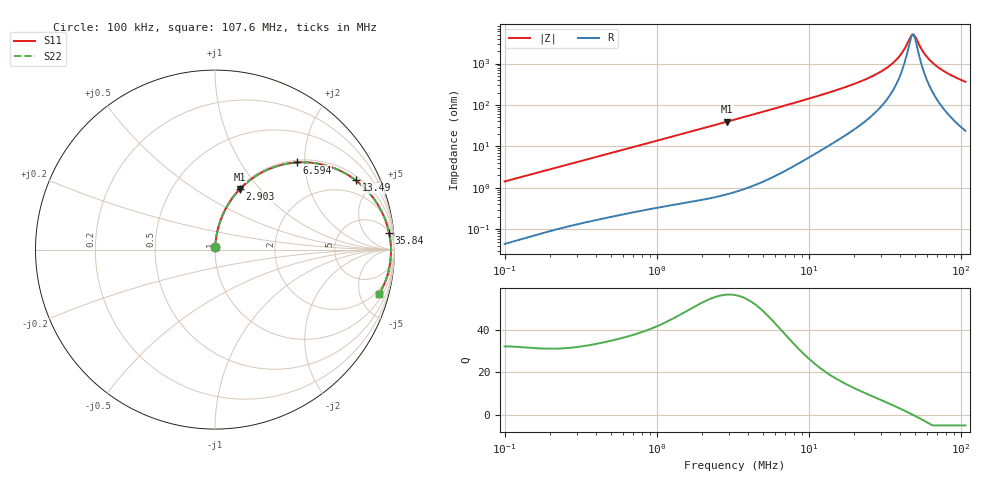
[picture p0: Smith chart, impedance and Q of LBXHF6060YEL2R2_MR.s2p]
! LBXHF6060YEL2R2_MR  S-PARAMETER MODEL  ( General Type )
! Model Generated by TAIYO YUDEN Corporation (http://www.ty-top.com)
! Version 1.0
! TAIYO YUDEN Control No. 200120NI43SB-FBB
! Copyright(c) 2020 TAIYO YUDEN CO.,LTD. All Rights Reserved.
! Product Description (link to TY-COMPAS)
! https://ds.yuden.co.jp/TYCOMPAS/or/detail?pn=LBXHF6060YEL2R2NMR&u=M
! Products Name : Inductors
! Characteristics :
!  Inductance : 2.2 uH , SRF(min) : 36 MHz , DC Resistance(max) : 0.023 Ohm
!  Rated Current : Saturation :8500 mA , Temp Rise : 3000 mA
!  Case Size : 6.0 x 6.0 / 0.236 x 0.236 [mm/inch] , Thickness : 4.5 / 0.177 [mm/inch]
!  (Conditions: Temperature = 25 degC , DC Bias Current/Voltage = 0A / 0V)
! External Node Assignments :
!  1  o---GGG---o  2
! GND o---------o GND
! Frequency Range : 0.1MHz  -  107.617193MHz  [ 402 STEP ]
# MHz S RI R 50
! Freq[MHz].  S11 Real  S11 Imag  S21 Real  S21 Imag  S12 Real  S12 Imag  S22 Real  S22 Imag
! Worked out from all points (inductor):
!   401 points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, 100 kHz to 107.6 MHz, reference 50 ohm
!   read as one part in series: L = 2.27 uH near 103.6 kHz
!   highest Q = 56.4 at 2.903 MHz (marker M1), where L = 2.17 uH
!   self-resonance near 48.22 MHz
!   S11 on the Smith chart (normalised r, x): 100 kHz: 1.00, +0.03; 2.903 MHz: 1.01, +0.79; 6.594 MHz: 1.05, +1.82; 13.49 MHz: 1.21, +3.95; 35.84 MHz: 5, +20; 107.6 MHz: 1.48, -7.26
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0.1  0.00065 0.0143  0.9994 -0.0143  0.9994 -0.0143  0.00065 0.0143
0.321988  0.00341 0.0448  0.9966 -0.0448  0.9966 -0.0448  0.00341 0.0448
1.036765  0.0229 0.1382  0.9771 -0.1382  0.9771 -0.1382  0.0229 0.1382
1.844211  0.0633 0.2341  0.9367 -0.2341  0.9367 -0.2341  0.0633 0.2341
2.90324  0.1395 0.3378  0.8605 -0.3378  0.8605 -0.3378  0.1395 0.3378
3.280506  0.1709 0.3677  0.8291 -0.3677  0.8291 -0.3677  0.1709 0.3677
4.570411  0.2851 0.4418  0.7149 -0.4418  0.7149 -0.4418  0.2851 0.4418
6.593697  0.4552 0.4856  0.5448 -0.4856  0.5448 -0.4856  0.4552 0.4856
10.56285  0.6866 0.4443  0.3134 -0.4443  0.3134 -0.4443  0.6866 0.4443
13.48643  0.7845 0.386  0.2155 -0.386  0.2155 -0.386  0.7845 0.386
23.57477  0.9255 0.2181  0.0745 -0.2181  0.0745 -0.2181  0.9255 0.2181
29.06724  0.9533 0.1538  0.0467 -0.1538  0.0467 -0.1538  0.9533 0.1538
34.01114  0.9673 0.1062  0.0327 -0.1062  0.0327 -0.1062  0.9673 0.1062
35.83936  0.9708 0.0905  0.0292 -0.0905  0.0292 -0.0905  0.9708 0.0905
41.20956  0.9775 0.0489  0.0225 -0.0489  0.0225 -0.0489  0.9775 0.0489
47.38442  0.9805 0.00736  0.0195 -0.00736  0.0195 -0.00736  0.9805 0.00736
49.06762  0.9807 -0.00303  0.0193 0.00303  0.0193 0.00303  0.9807 -0.00303
50.81061  0.9806 -0.0134  0.0194 0.0134  0.0194 0.0134  0.9806 -0.0134
57.41327  0.9786 -0.05  0.0214 0.05  0.0214 0.05  0.9786 -0.05
66.01611  0.9728 -0.0924  0.0272 0.0924  0.0272 0.0924  0.9728 -0.0924
81.39662  0.9561 -0.1574  0.0439 0.1574  0.0439 0.1574  0.9561 -0.1574
107.6172  0.9158 -0.2468  0.0842 0.2468  0.0842 0.2468  0.9158 -0.2468
